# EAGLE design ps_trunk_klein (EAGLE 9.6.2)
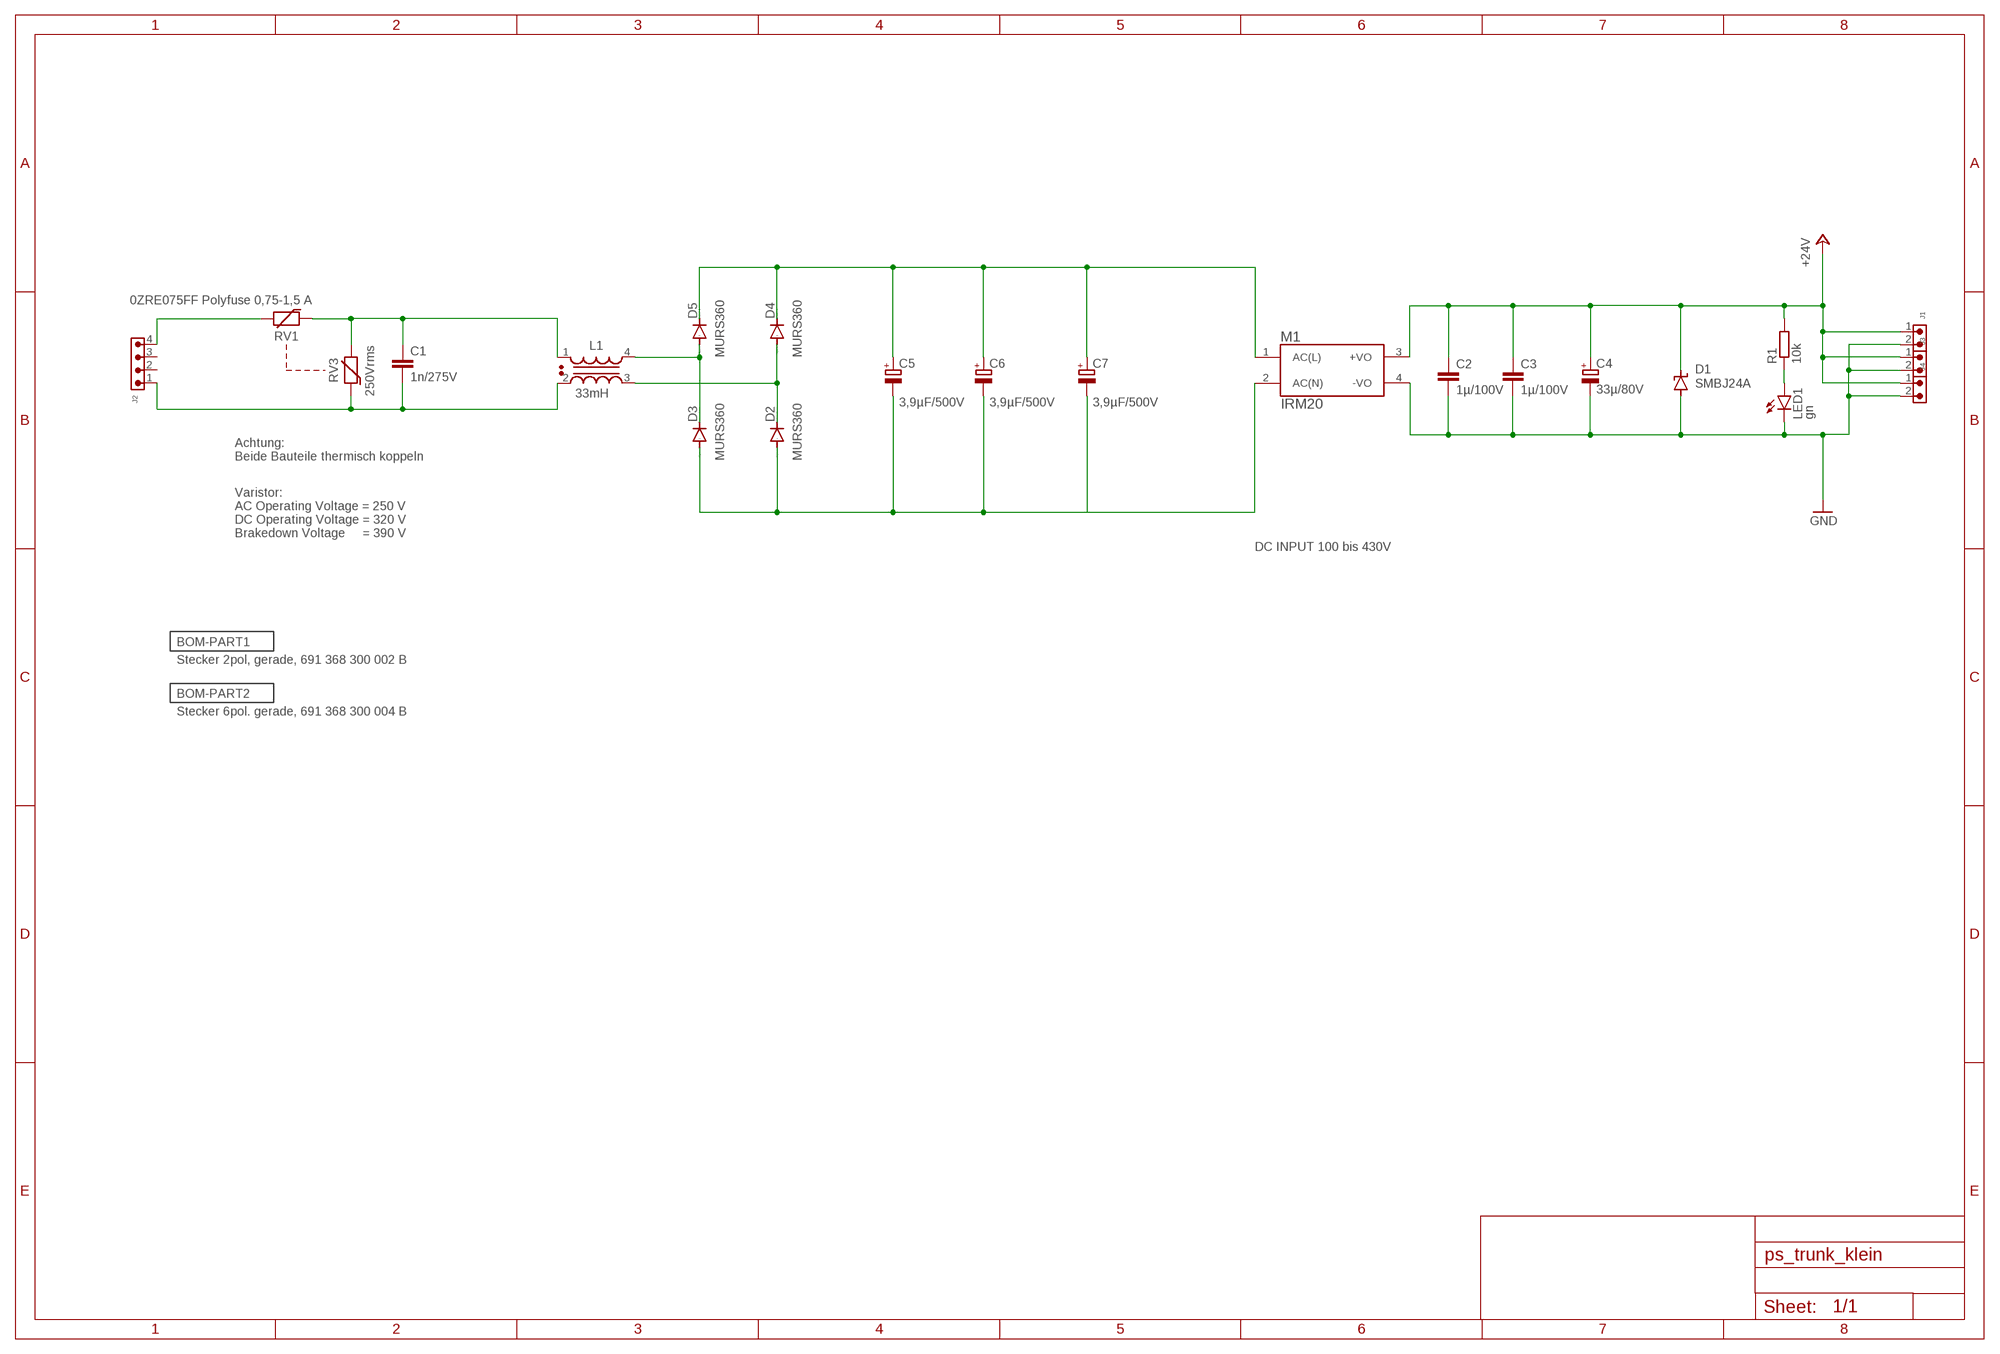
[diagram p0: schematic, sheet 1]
BOM-PART1 (BOM-PART): BOM: INCLUDE; QTY: 3
BOM-PART2 (BOM-PART): BOM: INCLUDE; QTY: 1

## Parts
C1  1n/275V  C-EU150-054X183  [C150-054X183]
C2  1µ/100V  C-EUC1210  [C1210]
C3  1µ/100V  C-EUC1210  [C1210]
C4  33µ/80V  CPOL-EUG  [PANASONIC_G]
C5  3,9µF/500V  CPOL-EUG  [PANASONIC_G]
C6  3,9µF/500V  CPOL-EUG  [PANASONIC_G]
C7  3,9µF/500V  CPOL-EUG  [PANASONIC_G]
D1  SMBJ24A  SUPPRESSOR-SMBJ  [SMBJ]
D2  MURS360  DIODE-SMC  [SMC]
D3  MURS360  DIODE-SMC  [SMC]
D4  MURS360  DIODE-SMC  [SMC]
D5  MURS360  DIODE-SMC  [SMC]
J1  691322310002  [691322310002]
J2  691322310004  [691322310004]
J3  691322310002  [691322310002]
J4  691322310002  [691322310002]
L1  33mH  WE-CMBNC_M_7448030333  [WE-CMBNC_M_7448030333]
LED1  gn  LEDCHIP-LED0603  [CHIP-LED0603]
M1  IRM20  [IRM-20]
R1  10k  R-EU_R0603  [R0603]
RV1  0ZRE075FF Polyfuse 0,75-1,5 A  WE-VD_10MM_820512511  [WE-VD_10MM_820512511]
RV3  250Vrms  WE-VD_10MM_820512511  [WE-VD_10MM_820512511]

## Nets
+24V: C2.1 C3.1 C4.+ D1.C J1.1 J3.1 J4.1 M1.3(+VO) R1.2
GND: C2.2 C3.2 C4.- D1.A J1.2 J3.2 J4.2 LED1.C M1.4(-VO)
N$1: J2.4 RV1.2
N$2: C1.2 J2.1 L1.2 RV3.1
N$3: C1.1 L1.1 RV1.1 RV3.2
N$4: LED1.A R1.1
N$5: D3.C D5.A L1.4
N$6: D2.C D4.A L1.3
N$8: C5.+ C6.+ C7.+ D4.C D5.C M1.1(AC(L))
N$9: C5.- C6.- C7.- D2.A D3.A M1.2(AC(N))
Unconnected: J2.2 J2.3

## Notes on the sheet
- Achtung:
  Beide Bauteile thermisch koppeln
- Varistor:
  AC Operating Voltage = 250 V
  DC Operating Voltage = 320 V 
  Brakedown Voltage     = 390 V
- DC INPUT 100 bis 430V

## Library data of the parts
C1-C3 = rcl:C-EU: CAPACITOR, European symbol; SPICEPREFIX: C
C4-C7 = rcl:CPOL-EU: POLARIZED CAPACITOR, European symbol; SPICEPREFIX: C
D1 = diode:SUPPRESSOR-: Suppressor diode
D2-D5 = diode:DIODE-: DIODE
J1 J3 J4 = Wurth_Connectors_WR-TBL Pluggable Connector:691322310002: WR-TBL Serie 322 - 3.81 mm Horizontal PCB Header; DATASHEET-URL: https://www.we-online.com/catalog/datasheet/691322310002.pdf; IR-UL: 10A; IR-VDE: 10.5A; MOUNT: THT; PART-NUMBER: 691322310002; PINS: 2; PITCH: 3.81mm; TYPE: Horizontal; WORKING-VOLTAGE-UL: 300V (AC); WORKING-VOLTAGE-VDE: 300V (AC)
J2 = Wurth_Connectors_WR-TBL Pluggable Connector:691322310004: WR-TBL Serie 322 - 3.81 mm Horizontal PCB Header KIND PROPERTIES Pitch 3.81 mm MATERIAL PROPERTIES Insulator Material PA66 Insulator Flammability Rating UL94 V-0 Contact Material Brass Contact Plating Tin GENERAL INFORMATION Operating Temperature -40 up to +105 °C Compliance RoHS ELECTRICAL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; DATASHEET-URL: https://www.we-online.com/catalog/datasheet/691322310004.pdf; IR-UL: 10A; IR-VDE: 10.5A; MOUNT: THT; PART-NUMBER: 691322310004; PINS: 4; PITCH: 3.81mm; TYPE: Horizontal; WORKING-VOLTAGE-UL: 300V (AC); WORKING-VOLTAGE-VDE: 300V (AC)
L1 = Wurth_EMC Components_WE-CMBNC:WE-CMBNC_M: WE-CMBNC Common Mode Power Line Choke Nanocrystalline Characteristics Very high permeability nanocrystalline core material Improved isolation through plastic case and winding spacer High and stable inductance values up to 150 °C High rated currents Broadband suppression Small size Frequency range: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; DATASHEET-URL: https://www.we-online.com/catalog/datasheet/7448030333.pdf; IR: 2.5A; MOUNT: THT; PART-NUMBER: 7448030333; RDC: 90mOhm; VR: 250 V (AC); VT: 1500 V (AC)
LED1 = led:LED: LED
M1 = PSK-30D-24:IRM20
R1 = rcl:R-EU_: RESISTOR, European symbol; SPICEPREFIX: R
RV1 = Wurth_EMC Components_WE-VD:WE-VD_10MM: WE-VD Disk Varistor; DATASHEET-URL: https://www.we-online.com/catalog/datasheet/820512511.pdf; ICLAMP: 25A; IPEAK: 2500A; MOUNT: THT; PART-NUMBER: 820512511; PDISS: 0.4W; VALUE: 250Vrms; VBR: 390V; VDC: 320Vdc; WMAX: 60J
RV3 = Wurth_EMC Components_WE-VD:WE-VD_10MM: WE-VD Disk Varistor; DATASHEET-URL: https://www.we-online.com/catalog/datasheet/820512511.pdf; ICLAMP: 25A; IPEAK: 2500A; MOUNT: THT; PART-NUMBER: 820512511; PDISS: 0.4W; VBR: 390V; VDC: 320Vdc; WMAX: 60J

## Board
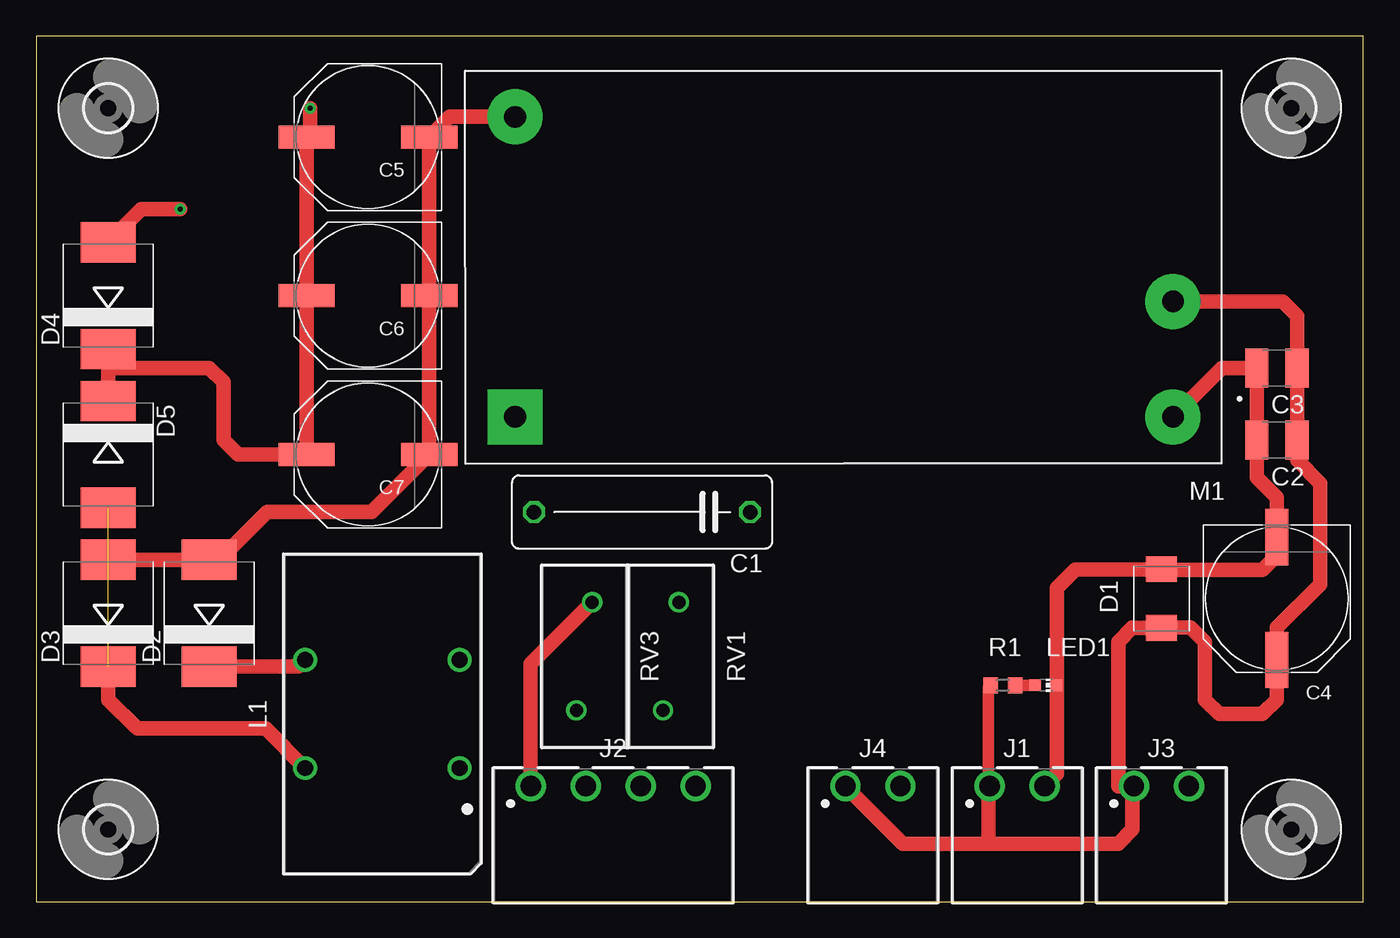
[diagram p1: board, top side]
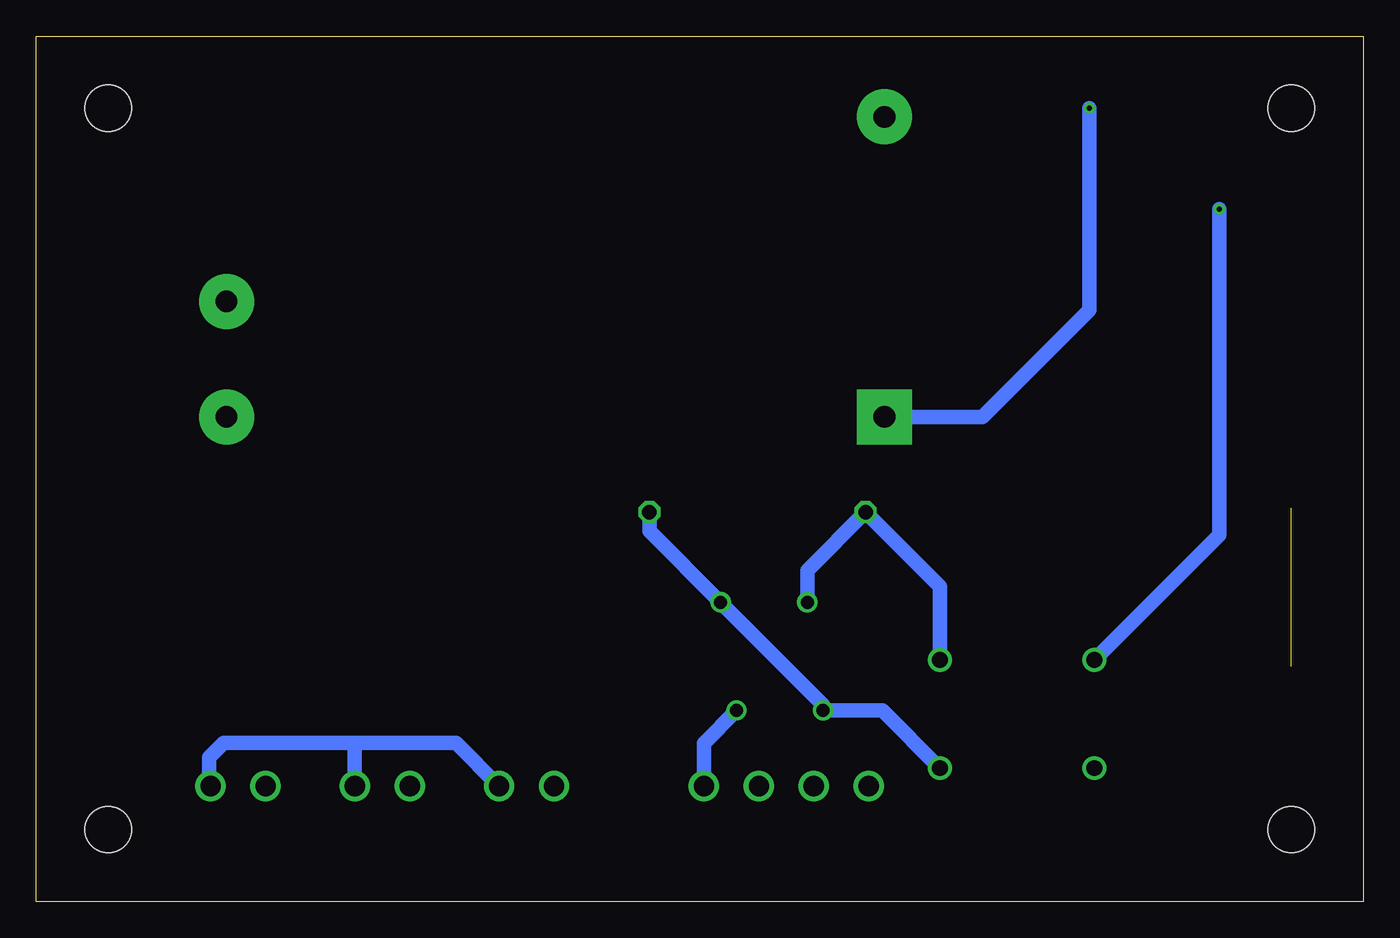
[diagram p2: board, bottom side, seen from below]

Size 92 x 60 mm. Coordinates in mm from the lower left corner, seen from the top.
Outline: 0,0 92,0 92,60 0,60 0,0
Copper layers (1*16): Top 0.035mm / dielectric 1.5mm / Bottom 0.035mm
Design rules "default": minimum track width 6mil, minimum drill 0.35mm, track to track 6mil, track to pad 6mil, pad to pad 6mil, via to via 6mil, smd to smd 6mil, copper to edge 40mil, drill to drill 6mil, minimum pad ring 10mil, minimum via ring 8mil, stop-mask expansion 4mil, vias tented up to drill 0mil, thermal gap 10mil

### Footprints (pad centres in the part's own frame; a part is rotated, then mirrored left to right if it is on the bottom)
C150-054X183 = drill 1.016 octagon: 1 -7.493,0; 2 7.493,0
C1210 = smd 1.6 x 2.7: 1 -1.4,0; 2 1.4,0
PANASONIC_G = smd 3.9 x 1.6: + 4.25,0; - -4.25,0
SMBJ = smd 1.78 x 2.16: A 2.04,0; C -2.03,0
SMC = smd 2.8 x 3.8: A 3.7,0; C -3.7,0
691322310002 = drill 1.4: 1 -1.905,0; 2 1.905,0
691322310004 = drill 1.4: 1 -5.715,0; 2 -1.905,0; 3 1.905,0; 4 5.715,0
WE-CMBNC_M_7448030333 = drill 1.1: 1 -3.75,-5.35; 2 3.75,-5.35; 3 3.75,5.35; 4 -3.75,5.35
CHIP-LED0603 = smd 0.8 x 0.8: A 0,-0.75; C 0,0.75
IRM-20 = drill 1.5 pad 3.81 square: 1 22.8,10.4 | drill 1.5 pad 3.81: 2 22.8,-10.4; 3 -22.8,2.4; 4 -22.8,10.4
R0603 = smd 1 x 1.1: 1 -0.85,0; 2 0.85,0
WE-VD_10MM_820512511 = drill 0.9: 1 -3.75,0.55; 2 3.75,-0.55
3,2 = hole 3.2: 0,0

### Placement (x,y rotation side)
C1  42,27 180 top
C2  86,32 180 top
C3  86,37 180 top
C4  86,21 270 top
C5  23,53 180 top
C6  23,42 180 top
C7  23,31 180 top
D1  78,21 90 top
D2  12,20 90 top
D3  5,20 90 top
D4  5,42 90 top
D5  5,31 270 top
J1  68,8 0 top
J2  40,8 0 top
J3  78,8 0 top
J4  58,8 0 top
L1  24,13 90 top
LED1  70,15 270 top
M1  56,44 180 top
R1  67,15 180 top
RV1  44,17 270 top
RV3  38,17 270 top
U$1  [3,2]  5,5 0 top
U$2  [3,2]  5,55 0 top
U$3  [3,2]  87,55 0 top
U$4  [3,2]  87,5 0 top

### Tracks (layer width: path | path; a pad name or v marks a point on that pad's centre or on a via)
+24V
  Top 0.813: R1.2 66,14.85 66,7.91
  Top 1.016: M1.3 86.4,41.6 87.4,40.6 C3.1 C2.1 87.4,30.6 89,29 89,22 86,19 C4.+ 86,14 85,13 82,13 81,14 81,18 80,19 78.03,19 D1.C 76.03,18.97 76,19 75,18 75,8 J3.1 76,7.91 76,5 75,4 66,4 | 66,4 66,7.91 J1.1 | J4.1 60.09,4 66,4
GND
  Top 1.016: M1.4 82.2,37 C3.2 C2.2 84.6,29.4 86,28 C4.- 86,24 85,23 78.04,23 D1.A 72.04,23.04 70.75,21.75 LED1.C 70.75,8.85 J1.2
  Bottom 1.016: J4.2 62.91,11 69.91,11 | J1.2 69.91,11 | 69.91,11 79,11 80,10 80,8.1 J3.2
N$1
  Bottom 1.016: J2.4 45.72,10.98 RV1.2
N$2
  Top 1.016: J2.1 34.28,16.48 RV3.1
  Bottom 1.016: RV3.1 38.55,22.96 C1.2 29.35,21.84 L1.2
N$3
  Bottom 1.016: C1.1 49.49,25.69 RV1.1 37.45,13.65 RV3.2 33.35,13.25 L1.1
N$4
  Top 0.813: LED1.A R1.1
N$5  (1 unrouted)
  Top 1.016: D3.C 5,14 7,12 15.9,12 L1.4
N$6  (via drill 0.35)
  Top 1.016: D2.C 18.2,16.3 L1.3 | D4.A 7.3,48 v10,48
  Bottom 1.016: v10,48 10,25.4 L1.3
N$8  (via drill 0.35)
  Top 1.016: D5.C 5,37 | 5,37 D4.C | 5,37 12,37 13,36 13,32 14,31 C7.+ C6.+ C5.+ 19,53.25 v19,55
  Bottom 1.016: M1.1 26.4,33.6 19,41 v19,55
N$9
  Top 1.016: D3.A D2.A 12.7,23 13,23 13,24 16,27 23.25,27 C7.- C6.- C5.- 28.65,54.4 M1.2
